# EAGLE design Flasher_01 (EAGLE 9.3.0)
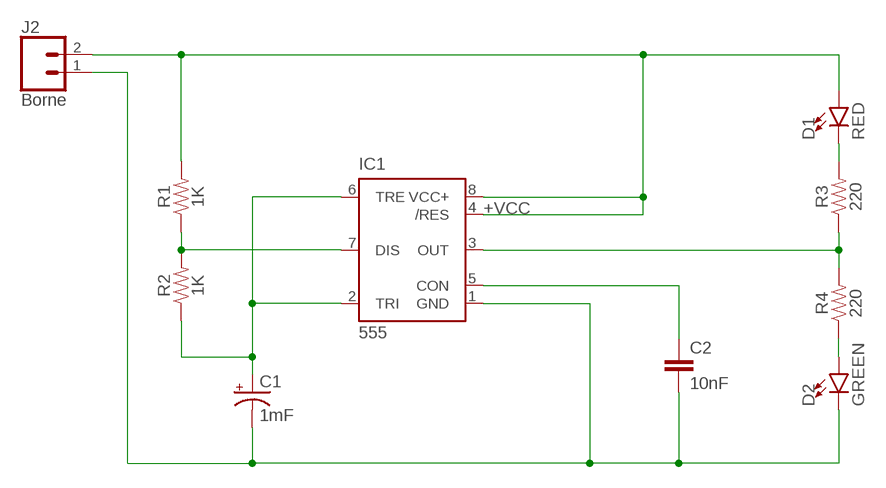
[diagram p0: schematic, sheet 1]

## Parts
C1  1mF  1000UF-RADIAL-5MM-25V-20%  [CPOL-RADIAL-5MM-10MM]
C2  10nF  10NF-0603-50V-10%  [0603]
D1  RED  LED5MM  [LED_5MM]
D2  GREEN  LED5MM  [LED_5MM]
IC1  555  555P  [DIP08]
J2  Borne  CONN_025MM  [SCREWTERMINAL-5MM-2]
R1  1K  10OHM-HORIZ-1/4W-1%  [AXIAL-0.3]
R2  1K  10OHM-HORIZ-1/4W-1%  [AXIAL-0.3]
R3  220  10OHM-HORIZ-1/4W-1%  [AXIAL-0.3]
R4  220  10OHM-HORIZ-1/4W-1%  [AXIAL-0.3]

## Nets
+VCC: D1.A IC1.4(/RES) IC1.8(VCC+) J2.2 R1.P$2
GND: C1.- C2.2 D2.K(C) IC1.1(GND) J2.1
N$1: D2.A R4.P$1
N$2: IC1.3(OUT) R3.P$1 R4.P$2
N$3: D1.K(C) R3.P$2
N$4: C2.1 IC1.5(CON)
N$6: IC1.7(DIS) R1.P$1 R2.P$2
N$8: C1.+ IC1.2(TRI) IC1.6(TRE) R2.P$1

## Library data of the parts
C1 = SparkFun-Capacitors:1000UF: 1,000µF/1mF ceramic capacitors; PROD_ID: CAP-09538
C2 = SparkFun-Capacitors:10NF: 0.01uF/10nF/10,000pF ceramic capacitors; PROD_ID: CAP-00867
D1 D2 = SparkFun-LED:LED: LED (Generic)
IC1 = SparkFun-IC-Special-Function:555: General purpose bipolar Timer Datasheet SparkFun Products SparkFun SparkPunk Sequencer Kit (KIT-12707) Storefront Component: 555 Timer (COM-09273) Two parts valid for production: VFP: IC-11930 (M7555 PTH) VFP: IC-09173 (555 PTH) - Preferred; PROD_ID: IC-09173; PROD_ID_ALT: IC-09173
J2 = SparkFun-Connectors:CONN_02: Multi connection point. Often used as Generic Header-pin footprint for 0.1 inch spaced/style header connections; SF_SKU: PRT-08432
R1-R4 = SparkFun-Resistors:10OHM: 10Ω resistor; PROD_ID: RES-12180; VALUE: 10

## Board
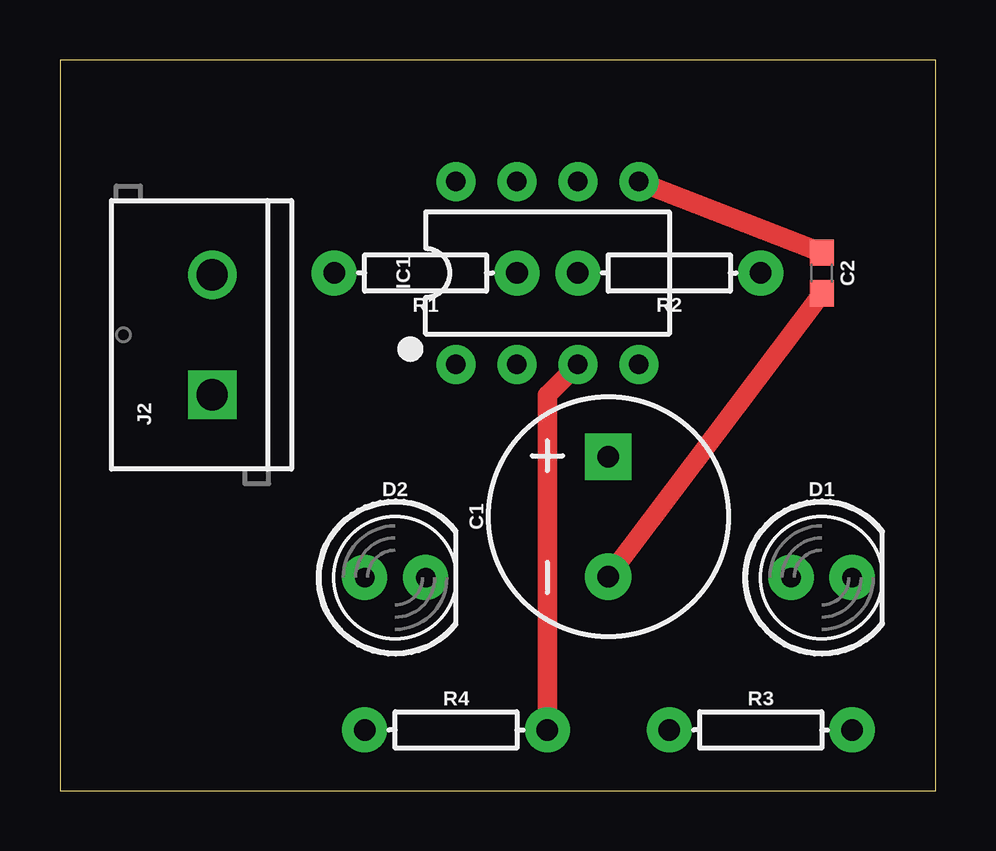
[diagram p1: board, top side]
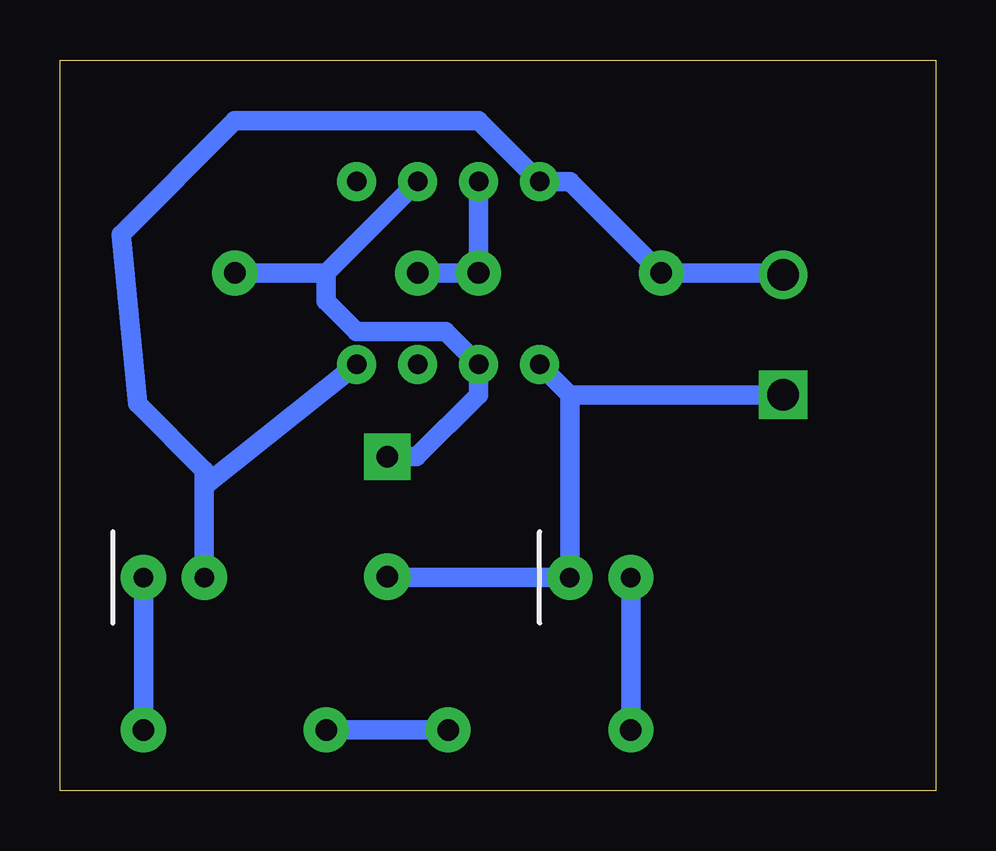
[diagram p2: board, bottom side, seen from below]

Size 36.5 x 30.47 mm. Coordinates in mm from the lower left corner, seen from the top.
Outline: 0,0 36.5,0 36.5,30.47 0,30.47 0,0
Copper layers (1*16): Top 0.035mm / dielectric 1.5mm / Bottom 0.035mm
Design rules "default": minimum track width 6mil, minimum drill 0.35mm, track to track 6mil, track to pad 6mil, pad to pad 6mil, via to via 6mil, smd to smd 6mil, copper to edge 40mil, drill to drill 6mil, minimum pad ring 10mil, minimum via ring 8mil, stop-mask expansion 4mil, vias tented up to drill 0mil, thermal gap 10mil

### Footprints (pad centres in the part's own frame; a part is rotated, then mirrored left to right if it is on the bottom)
CPOL-RADIAL-5MM-10MM = drill 0.9 pad 1.93 square: + 2.5,0 | drill 0.9 pad 1.93: - -2.5,0
0603 = smd 1.1 x 1: 1 -0.85,0; 2 0.85,0
LED_5MM = drill 0.813 pad 1.88: A -1.27,0; K 1.27,0
DIP08 = drill 0.813 pad 1.626: 1 -3.81,-3.81; 2 -1.27,-3.81; 3 1.27,-3.81; 4 3.81,-3.81; 5 3.81,3.81; 6 1.27,3.81; 7 -1.27,3.81; 8 -3.81,3.81
SCREWTERMINAL-5MM-2 = drill 1.3 pad 2.032 square: 1 0,0 | drill 1.3 pad 2.032: 2 5,0
AXIAL-0.3 = drill 0.9 pad 1.88: P$1 -3.81,0; P$2 3.81,0

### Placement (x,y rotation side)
C1  22.86,11.43 90 top
C2  31.75,21.59 270 top
D1  31.75,8.89 0 top
D2  13.97,8.89 0 top
IC1  20.32,21.59 0 top
J2  6.35,16.51 90 top
R1  15.24,21.59 180 top
R2  25.4,21.59 180 top
R3  29.21,2.54 0 top
R4  16.51,2.54 0 top

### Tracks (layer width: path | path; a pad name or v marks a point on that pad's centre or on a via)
+VCC
  Bottom 0.813: D1.A 30.48,12.7 | 30.48,12.7 30.48,13.36 33.27,16.15 33.95,23.2 29.21,27.94 19.05,27.94 IC1.8 15.24,25.4 R1.P$2 6.43,21.59 J2.2 | IC1.4 30.48,12.7
GND
  Top 0.813: C2.2 C1.-
  Bottom 0.813: C1.- 22.82,8.89 D2.K 15.24,16.51 | IC1.1 15.24,16.51 | J2.1 15.24,16.51
N$1
  Bottom 0.813: R4.P$1 D2.A
N$2
  Top 0.813: IC1.3 20.32,16.51 R4.P$2
  Bottom 0.813: R3.P$1 R4.P$2
N$3
  Bottom 0.813: D1.K R3.P$2
N$4
  Top 0.813: IC1.5 C2.1
N$6
  Bottom 0.813: R2.P$2 R1.P$1 IC1.7
N$8
  Bottom 0.813: C1.+ 21.63,13.93 19.05,16.51 IC1.2 20.42,19.15 24.13,19.15 25.4,20.42 25.4,21.59 | IC1.6 25.4,21.59 | 25.4,21.59 R2.P$1

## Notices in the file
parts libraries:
SparkFun-IC-Special-Function: Licensing: Creative Commons ShareAlike 4.0 International - https://creativecommons.org/licenses/by-sa/4.0
